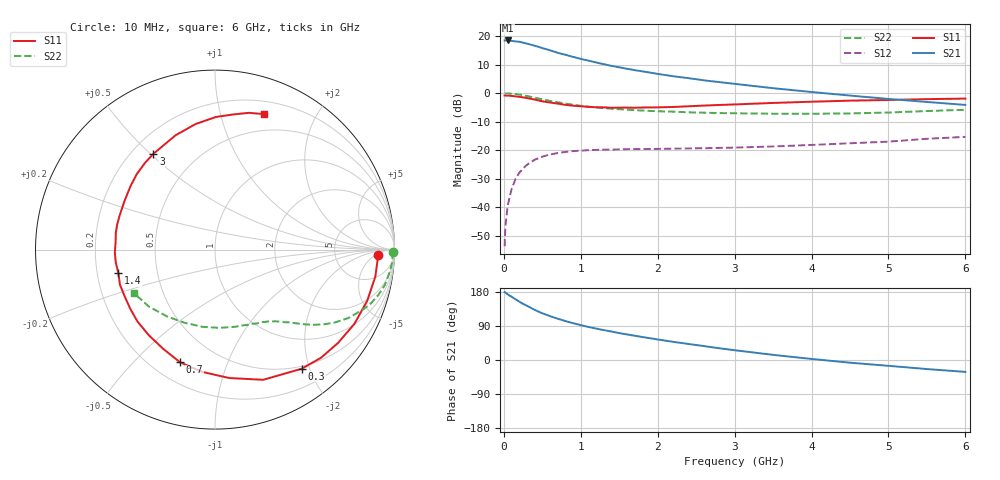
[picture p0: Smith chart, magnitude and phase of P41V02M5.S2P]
! SIEMENS Small Signal Semiconductors
! BFP182
! Si NPN RF Bipolar Junction Transistor in SOT143
! VCE = 1 V  IC = 2.5 mA
! Common Emitter S-Parameters:  March  1996
# GHz  S  MA  R  50
!  f  S11  S21  S12  S22
! GHz  MAG  ANG  MAG  ANG  MAG  ANG  MAG  ANG
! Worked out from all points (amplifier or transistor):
!   36 points, 10 MHz to 6 GHz, reference 50 ohm
!   highest |S21| = 18.4 dB at 50 MHz (marker M1)
!   |S21| within 3 dB of that: start of sweep to 543.5 MHz
!   unconditionally stable (mu >= 1): 1.951 GHz to end of sweep
!   at 250 MHz: K = 0.15, MSG = 22.0 dB, |S12| = -26.4 dB
!   at 1.4 GHz: K = 0.77, MSG = 14.7 dB, |S12| = -19.8 dB
!   at 6 GHz: K = 1.07, MAG = 4.0 dB, |S12| = -15.3 dB
!   S11 on the Smith chart (normalised r, x): 10 MHz: 19, -6; 300 MHz: 0.46, -1.88; 700 MHz: 0.31, -0.69; 1.4 GHz: 0.29, -0.11; 3 GHz: 0.29, +0.51; 6 GHz: 0.32, +1.38
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0.01  0.9089 -1.9  8.348 179.0  0.0021 85.1  0.9945 -0.8
0.02  0.9074 -3.9  8.327 178.0  0.0046 91.5  0.9891 -1.6
0.05  0.9059 -9.6  8.359 173.4  0.0108 88.0  0.991 -4.0
0.1  0.8946 -18.6  8.217 166.9  0.0207 77.9  0.9788 -8.0
0.2  0.8607 -37.1  7.937 154.1  0.0404 69.0  0.9448 -15.5
0.25  0.8437 -45.6  7.63 148.2  0.0481 64.3  0.9191 -19.0
0.3  0.8213 -53.9  7.348 143.2  0.0557 60.1  0.8913 -21.9
0.4  0.7734 -69.7  6.775 132.3  0.0682 52.4  0.8357 -27.1
0.5  0.7199 -83.7  6.151 123.3  0.0774 45.6  0.7804 -31.4
0.6  0.6847 -96.1  5.628 115.8  0.0845 40.6  0.7323 -34.7
0.7  0.6575 -107.2  5.084 109.0  0.0894 36.2  0.6925 -37.2
0.8  0.6236 -117.6  4.69 102.8  0.0936 32.4  0.6574 -39.4
0.9  0.6033 -127.5  4.322 97.2  0.0969 29.5  0.6269 -41.2
1.1  0.5754 -145.3  3.711 87.2  0.1005 25.0  0.5795 -44.4
1.4  0.554 -166.3  3.005 75.0  0.1029 19.7  0.5344 -48.6
1.8  0.5607 170.2  2.407 60.6  0.1053 16.7  0.4964 -53.8
2.2  0.5724 151.7  1.979 48.0  0.1069 14.8  0.4743 -60.1
3  0.6345 122.8  1.456 25.8  0.1115 14.1  0.4443 -75.4
3.5  0.6739 109.0  1.221 13.6  0.1167 14.1  0.4368 -86.7
4.5  0.7389 89.6  0.907 -7.1  0.1328 14.0  0.4418 -112.7
5.5  0.7854 76.0  0.701 -23.9  0.159 12.5  0.4864 -139.1
6  0.8028 70.0  0.623 -31.4  0.1718 9.2  0.5118 -151.7
